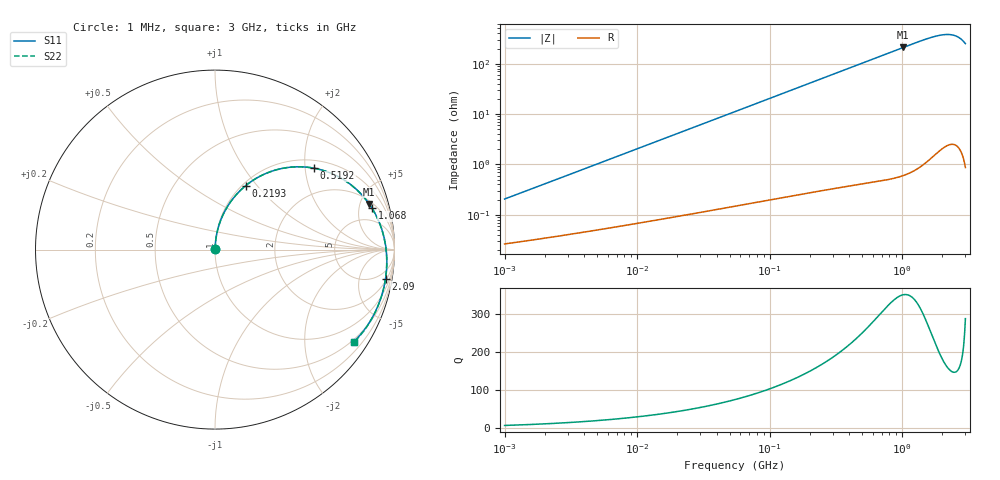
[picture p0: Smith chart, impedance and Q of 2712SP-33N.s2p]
# MHz  S  MA  R  50
!Freq  MagS11  AngS11  MagS21  AngS21  MagS12  AngS12  MagS22  AngS22
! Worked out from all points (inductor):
!   801 points, 1 MHz to 3 GHz, reference 50 ohm
!   read as one part in series: L = 32.5 nH near 1.041 MHz
!   highest Q = 350 at 1.016 GHz (marker M1), where L = 32.9 nH
!   S11 on the Smith chart (normalised r, x): 1 MHz: 1.00, +0.00; 219.3 MHz: 1.04, +0.87; 519.2 MHz: 1.20, +2.23; 1.068 GHz: 2.63, +6.69; 2.09 GHz: 2, -11; 3 GHz: 0.44, -3.26
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1  0.001977 82.2  0.9997 -0.1  0.9997 -0.1  0.001977 82.2
3.829105  0.007516 86.1  0.9995 -0.5  0.9995 -0.5  0.007515 86.1
14.51587  0.02843 86.6  0.9988 -1.8  0.9988 -1.8  0.02843 86.6
30.16481  0.05898 85.3  0.9971 -3.7  0.9971 -3.7  0.05897 85.3
55.02866  0.1071 82.6  0.9928 -6.6  0.9928 -6.6  0.1071 82.6
120.2275  0.229 75.2  0.9713 -14.3  0.9713 -14.3  0.229 75.2
160.7668  0.3001 70.6  0.9516 -18.9  0.9516 -18.9  0.3 70.6
208.6098  0.378 65.5  0.9233 -24.1  0.9233 -24.1  0.3779 65.5
219.327  0.3945 64.4  0.9163 -25.2  0.9163 -25.2  0.3944 64.4
278.9507  0.4794 58.5  0.8749 -31.2  0.8749 -31.2  0.4792 58.5
358.3557  0.5748 51.4  0.8155 -38.3  0.8155 -38.3  0.5745 51.4
519.181  0.7143 39.4  0.6972 -50.3  0.6972 -50.3  0.7138 39.4
640.7663  0.784 32.3  0.6182 -57.5  0.6182 -57.5  0.7835 32.3
790.8254  0.8426 25.0  0.5363 -64.8  0.5363 -64.8  0.8419 25.0
1015.938  0.8961 16.5  0.4418 -73.3  0.4418 -73.3  0.8953 16.5
1068.132  0.9047 14.8  0.424 -75.0  0.424 -75.0  0.9039 14.8
1516.793  0.9479 2.8  0.3154 -87.0  0.3154 -87.0  0.9472 2.8
2090.131  0.964 -9.8  0.2577 -99.4  0.2577 -99.4  0.9636 -9.8
2310.405  0.9637 -14.6  0.2556 -104.2  0.2556 -104.2  0.9637 -14.6
2528.433  0.9599 -19.7  0.2661 -109.3  0.2661 -109.3  0.9603 -19.7
2739.449  0.9512 -25.3  0.2914 -114.8  0.2914 -114.8  0.9522 -25.3
3000  0.9285 -33.6  0.3514 -123.3  0.3514 -123.3  0.9306 -33.6
